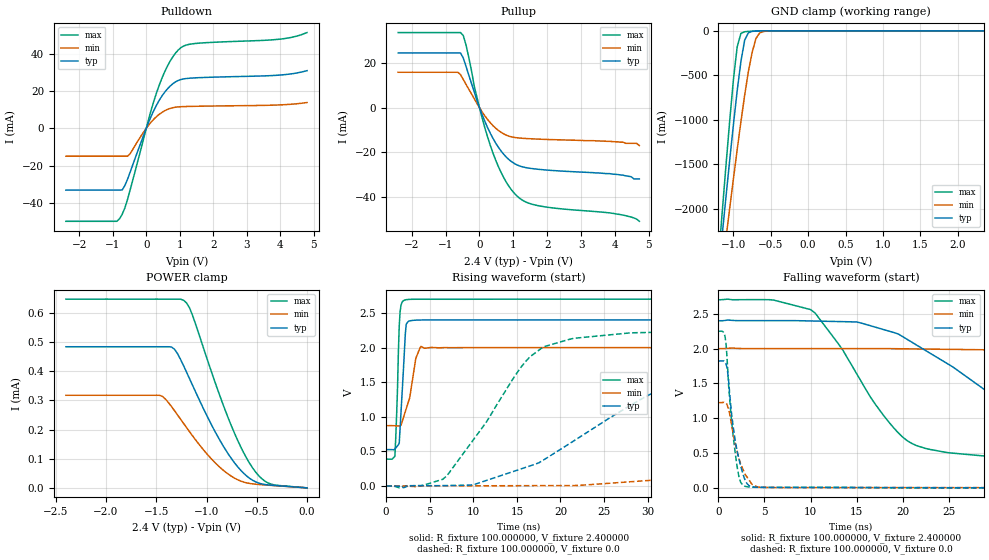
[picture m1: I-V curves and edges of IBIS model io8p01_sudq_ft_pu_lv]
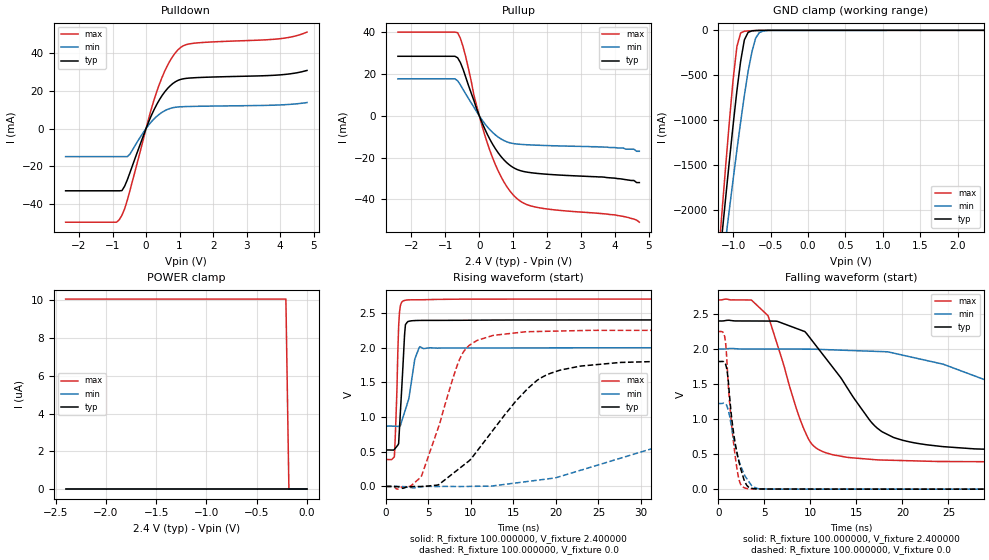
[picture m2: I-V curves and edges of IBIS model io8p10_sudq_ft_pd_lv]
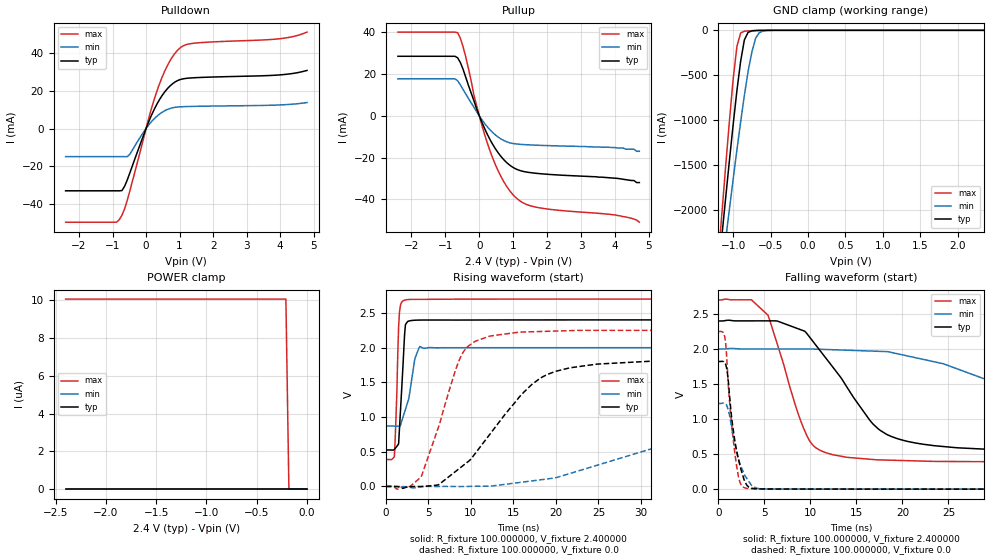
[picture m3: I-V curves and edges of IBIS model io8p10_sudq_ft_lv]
|   stm32f0_448_tssop20 IBIS Model
[IBIS ver]   4.2
[File name]  stm32f0_448_tssop20.ibs
[File Rev]   1.0
[Date]   15-5-2013
[Source] Data Created at STMicroelectronics
[Notes]   File originated from ELDO simulations.
[Disclaimer]  This information is for modeling purpose only and is
   not guaranted. The information is subject to change without
   notice.
[Copyright] Copyright 2015 STMicroelectronics Inc.
[Component] stm32f0_448_tssop20
[Manufacturer] STMicroelectronics
[Package]
| variable   typ   min   max
R_pkg   0.0   NA   NA
L_pkg   0.0H   NA   NA
C_pkg   0.0F   NA   NA
[Pin] signal_name  model_name   R_pin   L_pin   C_pin
1   BOOT0  vpp_test_hv
2   PF0   io8p_sudq_ft
3   PF1   io8p_sudq_ft
4   NRST   ioreset_tc_v33
5   VDDA   POWER
6   PA0   io8p_sudq_ft
7   PA1   io8p_sudq_ft
8   PA2   io8p_sudq_ft
9   PA3   io8p_sudq_ft
10   PA4   io8p_sudq_ft
11   PA5   io8p_sudq_ft
12   PA6   io8p_sudq_ft
13   PA7   io8p_sudq_ft
14   PB1   io8p_sudq_ft
15   VSS   GND
16   VDD   POWER
17   PA9   io8p_sudq_ft
18   PA10   io8p_sudq_ft
19   PA13   io8p_sudq_ft
20   PA14   io8p_sudq_ft
[Model Selector] io8p_sudq_ft
io8p01_sudq_ft_pd_lv  "SPEED01 2P0V, PD=40kOhm"
io8p01_sudq_ft_pu_lv  "SPEED01 2P0V, PU=40kOhm"
io8p01_sudq_ft_lv  "SPEED01 2P0V"
io8p10_sudq_ft_pd_lv  "SPEED10 2P0V, PD=40kOhm"
io8p10_sudq_ft_pu_lv  "SPEED10 2P0V, PU=40kOhm"
io8p10_sudq_ft_lv  "SPEED10 2P0V"
io8p11_sudq_ft_pd_lv  "SPEED11 2P0V, PD=40kOhm"
io8p11_sudq_ft_pu_lv  "SPEED11 2P0V, PU=40kOhm"
io8p11_sudq_ft_lv  "SPEED11 2P0V"
io8p01_sudq_ft_pd  "SPEED01, PD=40kOhm"
io8p01_sudq_ft_pu  "SPEED01, PU=40kOhm"
io8p01_sudq_ft  "SPEED01"
io8p10_sudq_ft_pd  "SPEED10, PD=40kOhm"
io8p10_sudq_ft_pu  "SPEED10, PU=40kOhm"
io8p10_sudq_ft  "SPEED10"
io8p11_sudq_ft_pd  "SPEED11, PD=40kOhm"
io8p11_sudq_ft_pu  "SPEED11, PU=40kOhm"
io8p11_sudq_ft  "SPEED11"
[Model Selector] ioreset_tc_v33
ioreset_tc_v33_pu_lv  "IORESET 2V + PU=40kOhm"
ioreset_tc_v33_nopu_lv  "IORESET 2V"
ioreset_tc_v33_pu  "IORESET + PU=40kOhm"
ioreset_tc_v33_nopu  "IORESET"
[Model Selector] vpp_test_hv
vpp_test_hv_3p3  "Input Buffer"
vpp_test_hv_2p4  "Input Buffer 2P0V"
| Models and submodels in the file (24): io8p01_sudq_ft_pd_lv (I/O), io8p01_sudq_ft_pu_lv (I/O), io8p01_sudq_ft_lv (I/O), io8p10_sudq_ft_pd_lv (I/O), io8p10_sudq_ft_pu_lv (I/O), io8p10_sudq_ft_lv (I/O), io8p11_sudq_ft_pd_lv (I/O), io8p11_sudq_ft_pu_lv (I/O), io8p11_sudq_ft_lv (I/O), io8p01_sudq_ft_pd (I/O), io8p01_sudq_ft_pu (I/O), io8p01_sudq_ft (I/O), io8p10_sudq_ft_pd (I/O), io8p10_sudq_ft_pu (I/O), io8p10_sudq_ft (I/O), io8p11_sudq_ft_pd (I/O), io8p11_sudq_ft_pu (I/O), io8p11_sudq_ft (I/O), ioreset_tc_v33_pu_lv (I/O_open_drain), ioreset_tc_v33_nopu_lv (I/O_open_drain), ioreset_tc_v33_pu (I/O_open_drain), ioreset_tc_v33_nopu (I/O_open_drain), vpp_test_hv_2p4 (Input), vpp_test_hv_3p3 (Input)
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|   Model io8p01_sudq_ft_pu_lv
[Model]  io8p01_sudq_ft_pu_lv
Model_type I/O
Polarity   Non-Inverting
Enable   Active-Low
Vinl =   0.720000V
Vinh =   1.680000V
Vmeas =  1.200000V
Cref =   50.000000pF
Rref =   100.000000M
Vref =   0.0V
C_comp   1.970100pF   1.887900pF   2.069400pF
[Temperature Range]   25.000000   0.125000k   -40.000000
[Pullup Reference]   2.400000V   2.000000V   2.700000V
[Pulldown Reference]   0.0V   0.0V   0.0V
[POWER Clamp Reference]   2.400000V   2.000000V   2.700000V
[GND Clamp Reference]   0.0V   0.0V   0.0V
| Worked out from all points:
|   slope of the pulldown table from 0 to 0.36 V, typ, clamps not added: 25.5 ohm
|   slope of the pullup table from 0 to 0.36 V, typ, clamps not added: 28.4 ohm
|   GND clamp passes 1 mA (typ) near -0.64 V on its own axis
|   rising waveform, R_fixture 100.000000, V_fixture 2.400000: 20-80 % time 497ps typ, 1.06ns min, 335ps max; typ from 0.527 V to 2.4 V
|   rising waveform, R_fixture 100.000000, V_fixture 0.0: 20-80 % time 14.6ns typ, 42.8ns min, 7.27ns max; typ from 0.001 V to 1.82 V
|   falling waveform, R_fixture 100.000000, V_fixture 2.400000: 20-80 % time 12.9ns typ, 32.5ns min, 7.06ns max; typ from 2.4 V to 0.527 V
|   falling waveform, R_fixture 100.000000, V_fixture 0.0: 20-80 % time 1.16ns typ, 1.4ns min, 913ps max; typ from 1.82 V to 0.001 V
[Pulldown]
|Voltage   I(typ)   I(min)   I(max)
-2.4V     -33.16mA   -14.98mA   -49.86mA
-880mV    -33.16mA   -14.98mA   -49.86mA
-800mV    -33.16mA   -14.98mA   -48.55mA
-640mV    -30.75mA   -14.98mA   -42.77mA
-480mV    -23.43mA   -13.57mA   -32.92mA
80mV      3.651mA    1.905mA    5.506mA
400mV     15.37mA    7.665mA    23.73mA
720mV     22.75mA    10.69mA    36.23mA
1.04V     26.18mA    11.57mA    43.27mA
1.52V     27.09mA    11.81mA    45.55mA
4V        28.55mA    12.55mA    47.81mA
4.8V      30.9mA     13.81mA    51.31mA
[Pullup]
|Voltage   I(typ)   I(min)   I(max)
-2.4V     24.57mA    15.91mA    33.73mA
-640mV    24.57mA    15.91mA    33.73mA
-480mV    22.32mA    12.71mA    32.43mA
-400mV    18.71mA    10.52mA    28.28mA
-160mV    7.421mA    4.162mA    10.02mA
0V        81fA       15.2pA     0A
320mV     -11.51mA   -6.781mA   -16.98mA
720mV     -21mA      -11.8mA    -31.53mA
1.2V      -26.24mA   -13.65mA   -40.83mA
1.76V     -27.69mA   -14.12mA   -44.07mA
3.84V     -29.6mA    -15.1mA    -47.2mA
4.72V     -32mA      -17mA      -51mA
[GND_clamp]
|Voltage   I(typ)   I(min)   I(max)
-2.4V     -9.788A    -9.782A    -9.734A
-1.2V     -2.718A    -3.02A     -2.568A
-1.15V    -2.29A     -2.675A    -2.036A
-1.1V     -1.868A    -2.333A    -1.515A
-1.05V    -1.454A    -1.995A    -1.012A
-950mV    -674.5mA   -1.337A    -180.5mA
-900mV    -345.2mA   -1.023A    -29.72mA
-850mV    -106.4mA   -726mA     -10.13mA
-750mV    -6.396mA   -244mA     -4.026mA
-700mV    -2.558mA   -88.61mA   -2.329mA
-600mV    -416uA     -7.739mA   -368uA
2.35V     0A         0A         0A
[POWER_clamp]
|Voltage   I(typ)   I(min)   I(max)
-2.4V     483.8uA    317.4uA    647uA
-1.47V    483.8uA    317.4uA    647uA
-1.32V    475.6uA    265.2uA    647uA
-1.23V    419.7uA    221.6uA    643.3uA
-1.17V    374.8uA    192.7uA    617.6uA
-1.14V    352.1uA    178.7uA    591.9uA
-840mV    147uA      62.15uA    289.6uA
-690mV    72.24uA    27.76uA    162.7uA
-540mV    25.74uA    13.55uA    67.63uA
-450mV    13.38uA    10.75uA    31.36uA
-360mV    9.231uA    8.535uA    12.97uA
0V        0A         0A         0A
[Ramp]
| variable   typ   min   max
dV/dt_r  1.09269/14.55881n   0.73353/42.71845n   1.34908/7.26325n
dV/dt_f  1.12400/12.83842n   0.67649/32.44923n   1.38689/7.04961n
R_load = 100.000000
[Rising Waveform]
R_fixture= 100.000000
V_fixture= 2.400000
V_fixture_min= 2.000000
V_fixture_max= 2.700000
|time   V(typ)   V(min)   V(max)
0s        526.5mV    872.5mV    388.6mV
1.001ns   534.8mV    870.7mV    429.3mV
1.301ns   581.8mV    869.1mV    1.401V
1.502ns   620.7mV    868.5mV    2.316V
1.602ns   841mV      868.2mV    2.522V
2.102ns   1.968V     1.038V     2.685V
2.302ns   2.337V     1.118V     2.692V
3.403ns   2.396V     1.846V     2.698V
4.004ns   2.398V     2.018V     2.698V
49.85ns   2.4V       2V         2.7V
[Rising Waveform]
R_fixture= 100.000000
V_fixture= 0.0
V_fixture_min= 0.0
V_fixture_max= 0.0
|time   V(typ)   V(min)   V(max)
0s        1.057mV    1.357mV    941.6uV
6.507ns   6.739mV    4.851mV    98.8mV
15.52ns   249.4mV    5.766mV    1.725V
18.02ns   374.6mV    6.657mV    2.009V
28.03ns   1.166V     62.6mV     2.213V
34.53ns   1.553V     120.9mV    2.23V
43.04ns   1.725V     229mV      2.248V
79.08ns   1.822V     883.8mV    2.25V
103.1ns   1.822V     1.116V     2.249V
249.2ns   1.822V     1.224V     2.25V
[Falling Waveform]
R_fixture= 100.000000
V_fixture= 2.400000
V_fixture_min= 2.000000
V_fixture_max= 2.700000
|time   V(typ)   V(min)   V(max)
0s        2.4V       2V         2.7V
10.01ns   2.397V     2V         2.56V
15.02ns   2.383V     2V         1.64V
20.02ns   2.171V     1.997V     729.2mV
29.53ns   1.353V     1.982V     451.1mV
38.04ns   762.8mV    1.926V     413.2mV
57.06ns   576.4mV    1.555V     391.8mV
84.58ns   537.8mV    1.049V     388.5mV
102.6ns   530.3mV    958.5mV    388.5mV
249.2ns   526.5mV    872.5mV    388.6mV
[Falling Waveform]
R_fixture= 100.000000
V_fixture= 0.0
V_fixture_min= 0.0
V_fixture_max= 0.0
|time   V(typ)   V(min)   V(max)
0s        1.822V     1.224V     2.25V
700.7ps   1.803V     1.224V     2.18V
800.8ps   1.785V     1.217V     2.098V
1.001ns   1.655V     1.167V     1.705V
1.401ns   1.091V     924.7mV    994.1mV
1.802ns   692.7mV    650.1mV    517.8mV
2.302ns   370.4mV    389.6mV    121.1mV
2.903ns   110.3mV    193.7mV    21.86mV
4.605ns   7.762mV    8.133mV    8.175mV
49.85ns   1.057mV    1.357mV    941.6uV
|   Model io8p10_sudq_ft_pd_lv
[Model]  io8p10_sudq_ft_pd_lv
Model_type I/O
Polarity   Non-Inverting
Enable   Active-Low
Vinl =   0.720000V
Vinh =   1.680000V
Vmeas =  1.200000V
Cref =   50.000000pF
Rref =   100.000000M
Vref =   0.0V
C_comp   1.970100pF   1.887900pF   2.069400pF
[Temperature Range]   25.000000   0.125000k   -40.000000
[Pullup Reference]   2.400000V   2.000000V   2.700000V
[Pulldown Reference]   0.0V   0.0V   0.0V
[POWER Clamp Reference]   2.400000V   2.000000V   2.700000V
[GND Clamp Reference]   0.0V   0.0V   0.0V
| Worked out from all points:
|   slope of the pulldown table from 0 to 0.36 V, typ, clamps not added: 25.5 ohm
|   slope of the pullup table from 0 to 0.36 V, typ, clamps not added: 28.4 ohm
|   GND clamp passes 1 mA (typ) near -0.64 V on its own axis
|   rising waveform, R_fixture 100.000000, V_fixture 2.400000: 20-80 % time 501ps typ, 1.06ns min, 337ps max; typ from 0.525 V to 2.4 V
|   rising waveform, R_fixture 100.000000, V_fixture 0.0: 20-80 % time 7.37ns typ, 21.8ns min, 3.53ns max; typ from 0 V to 1.82 V
|   falling waveform, R_fixture 100.000000, V_fixture 2.400000: 20-80 % time 6.27ns typ, 17.5ns min, 3.34ns max; typ from 2.4 V to 0.525 V
|   falling waveform, R_fixture 100.000000, V_fixture 0.0: 20-80 % time 1.15ns typ, 1.39ns min, 910ps max; typ from 1.82 V to 0 V
[Pulldown]
|Voltage   I(typ)   I(min)   I(max)
-2.4V     -33.16mA   -14.98mA   -49.86mA
-880mV    -33.16mA   -14.98mA   -49.86mA
-800mV    -33.16mA   -14.98mA   -48.55mA
-640mV    -30.75mA   -14.98mA   -42.76mA
-480mV    -23.43mA   -13.57mA   -32.92mA
80mV      3.651mA    1.905mA    5.506mA
400mV     15.37mA    7.665mA    23.73mA
720mV     22.75mA    10.69mA    36.23mA
1.04V     26.18mA    11.57mA    43.27mA
1.52V     27.09mA    11.81mA    45.55mA
4V        28.55mA    12.55mA    47.81mA
4.8V      30.9mA     13.81mA    51.31mA
[Pullup]
|Voltage   I(typ)   I(min)   I(max)
-2.4V     28.56mA    17.75mA    40.16mA
-720mV    28.56mA    17.75mA    40.16mA
-640mV    27.85mA    16.83mA    39.87mA
-480mV    22.39mA    12.66mA    33.22mA
-80mV     3.427mA    2.067mA    4.957mA
160mV     -6.219mA   -3.715mA   -9.137mA
320mV     -11.51mA   -6.781mA   -16.98mA
720mV     -21mA      -11.8mA    -31.53mA
1.12V     -25.77mA   -13.54mA   -39.82mA
1.76V     -27.69mA   -14.12mA   -44.07mA
4V        -29.9mA    -15.2mA    -47.5mA
4.72V     -32mA      -17mA      -51mA
[GND_clamp]
|Voltage   I(typ)   I(min)   I(max)
-2.4V     -9.788A    -9.782A    -9.734A
-1.2V     -2.718A    -3.021A    -2.568A
-1.15V    -2.29A     -2.675A    -2.036A
-1.1V     -1.868A    -2.333A    -1.515A
-1.05V    -1.454A    -1.995A    -1.012A
-950mV    -674.5mA   -1.337A    -180.6mA
-900mV    -345.2mA   -1.023A    -29.74mA
-850mV    -106.4mA   -726mA     -10.14mA
-750mV    -6.411mA   -244mA     -4.042mA
-700mV    -2.572mA   -88.62mA   -2.346mA
-600mV    -429.6uA   -7.75mA    -383.5uA
2.35V     59.77uA    46.33uA    66.89uA
[POWER_clamp]
|Voltage   I(typ)   I(min)   I(max)
-2.4V     0A         0A         10.06uA
-210mV    0A         0A         10.06uA
-180mV    0A         0A         0A
0V        0A         0A         0A
[Ramp]
| variable   typ   min   max
dV/dt_r  1.09206/7.36205n   0.73212/21.76780n   1.34880/3.52140n
dV/dt_f  1.12434/6.26286n   0.67629/17.46251n   1.38699/3.33301n
R_load = 100.000000
[Rising Waveform]
R_fixture= 100.000000
V_fixture= 2.400000
V_fixture_min= 2.000000
V_fixture_max= 2.700000
|time   V(typ)   V(min)   V(max)
0s        524.8mV    868.7mV    387.2mV
1.001ns   532.8mV    867mV      426.6mV
1.301ns   578.6mV    865.5mV    1.387V
1.502ns   616.5mV    864.9mV    2.303V
1.702ns   1.053V     875.4mV    2.602V
2.102ns   1.953V     1.031V     2.676V
2.302ns   2.331V     1.108V     2.683V
3.403ns   2.389V     1.835V     2.689V
4.004ns   2.392V     2.014V     2.689V
49.85ns   2.399V     1.999V     2.699V
[Rising Waveform]
R_fixture= 100.000000
V_fixture= 0.0
V_fixture_min= 0.0
V_fixture_max= 0.0
|time   V(typ)   V(min)   V(max)
0s        1.768nV    15.89nV    1.355nV
2.803ns   -3.26mV    -14.06mV   -1.551mV
4.204ns   -1.822mV   -2.484mV   153.2mV
6.206ns   24.43mV    -1.172mV   860.8mV
8.809ns   274.4mV    -1.373mV   1.867V
12.61ns   812.3mV    7.914mV    2.175V
17.82ns   1.532V     89.58mV    2.232V
23.02ns   1.735V     237.2mV    2.246V
50.05ns   1.82V      1.08V      2.248V
99.7ns    1.82V      1.221V     2.248V
[Falling Waveform]
R_fixture= 100.000000
V_fixture= 2.400000
V_fixture_min= 2.000000
V_fixture_max= 2.700000
|time   V(typ)   V(min)   V(max)
0s        2.399V     1.999V     2.699V
3.604ns   2.399V     1.998V     2.698V
5.405ns   2.398V     1.998V     2.475V
9.61ns    2.218V     1.997V     767.5mV
12.61ns   1.708V     1.986V     485.9mV
17.62ns   835.2mV    1.963V     416.1mV
24.42ns   606.3mV    1.782V     394.4mV
31.83ns   557.1mV    1.421V     389.7mV
47.25ns   529mV      987.2mV    387.3mV
99.7ns    524.8mV    868.7mV    387.2mV
[Falling Waveform]
R_fixture= 100.000000
V_fixture= 0.0
V_fixture_min= 0.0
V_fixture_max= 0.0
|time   V(typ)   V(min)   V(max)
0s        1.82V      1.221V     2.248V
700.7ps   1.8V       1.221V     2.179V
800.8ps   1.783V     1.214V     2.096V
1.001ns   1.653V     1.163V     1.703V
1.401ns   1.09V      921.9mV    991.5mV
1.802ns   688.2mV    647.3mV    514.6mV
2.302ns   364.8mV    386.2mV    116.7mV
2.903ns   104.8mV    188.7mV    16.24mV
4.705ns   2.13mV     3.846mV    2.055mV
49.85ns   1.768nV    15.89nV    1.355nV
|   Model io8p10_sudq_ft_lv
[Model]  io8p10_sudq_ft_lv
Model_type I/O
Polarity   Non-Inverting
Enable   Active-Low
Vinl =   0.720000V
Vinh =   1.680000V
Vmeas =  1.200000V
Cref =   50.000000pF
Rref =   100.000000M
Vref =   0.0V
C_comp   1.970100pF   1.887900pF   2.069400pF
[Temperature Range]   25.000000   0.125000k   -40.000000
[Pullup Reference]   2.400000V   2.000000V   2.700000V
[Pulldown Reference]   0.0V   0.0V   0.0V
[POWER Clamp Reference]   2.400000V   2.000000V   2.700000V
[GND Clamp Reference]   0.0V   0.0V   0.0V
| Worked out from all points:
|   slope of the pulldown table from 0 to 0.36 V, typ, clamps not added: 25.5 ohm
|   slope of the pullup table from 0 to 0.36 V, typ, clamps not added: 28.4 ohm
|   GND clamp passes 1 mA (typ) near -0.64 V on its own axis
|   rising waveform, R_fixture 100.000000, V_fixture 2.400000: 20-80 % time 501ps typ, 1.06ns min, 336ps max; typ from 0.525 V to 2.4 V
|   rising waveform, R_fixture 100.000000, V_fixture 0.0: 20-80 % time 7.32ns typ, 21.7ns min, 3.52ns max; typ from 0 V to 1.82 V
|   falling waveform, R_fixture 100.000000, V_fixture 2.400000: 20-80 % time 6.27ns typ, 18.5ns min, 3.33ns max; typ from 2.4 V to 0.525 V
|   falling waveform, R_fixture 100.000000, V_fixture 0.0: 20-80 % time 1.16ns typ, 1.4ns min, 914ps max; typ from 1.82 V to 0 V
[Pulldown]
|Voltage   I(typ)   I(min)   I(max)
-2.4V     -33.16mA   -14.98mA   -49.86mA
-880mV    -33.16mA   -14.98mA   -49.86mA
-800mV    -33.16mA   -14.98mA   -48.55mA
-640mV    -30.75mA   -14.98mA   -42.76mA
-480mV    -23.43mA   -13.57mA   -32.92mA
80mV      3.651mA    1.905mA    5.506mA
400mV     15.37mA    7.665mA    23.73mA
720mV     22.75mA    10.69mA    36.23mA
1.04V     26.18mA    11.57mA    43.27mA
1.52V     27.09mA    11.81mA    45.55mA
4V        28.55mA    12.55mA    47.81mA
4.8V      30.9mA     13.81mA    51.31mA
[Pullup]
|Voltage   I(typ)   I(min)   I(max)
-2.4V     28.57mA    17.75mA    40.17mA
-720mV    28.57mA    17.75mA    40.17mA
-640mV    27.85mA    16.83mA    39.88mA
-480mV    22.38mA    12.65mA    33.22mA
-80mV     3.427mA    2.066mA    4.957mA
160mV     -6.219mA   -3.715mA   -9.137mA
320mV     -11.51mA   -6.781mA   -16.98mA
720mV     -21mA      -11.8mA    -31.54mA
1.12V     -25.77mA   -13.54mA   -39.82mA
1.76V     -27.69mA   -14.12mA   -44.07mA
4V        -29.9mA    -15.2mA    -47.5mA
4.72V     -32mA      -17mA      -51mA
[GND_clamp]
|Voltage   I(typ)   I(min)   I(max)
-2.4V     -9.788A    -9.782A    -9.734A
-1.2V     -2.718A    -3.02A     -2.568A
-1.15V    -2.29A     -2.675A    -2.036A
-1.1V     -1.868A    -2.333A    -1.515A
-1.05V    -1.454A    -1.995A    -1.012A
-950mV    -674.5mA   -1.337A    -180.5mA
-900mV    -345.2mA   -1.023A    -29.72mA
-850mV    -106.4mA   -726mA     -10.13mA
-750mV    -6.396mA   -244mA     -4.026mA
-700mV    -2.558mA   -88.61mA   -2.329mA
-600mV    -416uA     -7.739mA   -368uA
2.35V     0A         0A         0A
[POWER_clamp]
|Voltage   I(typ)   I(min)   I(max)
-2.4V     0A         0A         10.06uA
-210mV    0A         0A         10.06uA
-180mV    0A         0A         0A
0V        0A         0A         0A
[Ramp]
| variable   typ   min   max
dV/dt_r  1.09308/7.31082n   0.73308/21.71145n   1.34964/3.51759n
dV/dt_f  1.12481/6.26349n   0.67631/18.49686n   1.38754/3.32485n
R_load = 100.000000
[Rising Waveform]
R_fixture= 100.000000
V_fixture= 2.400000
V_fixture_min= 2.000000
V_fixture_max= 2.700000
|time   V(typ)   V(min)   V(max)
0s        525.2mV    870.3mV    387.4mV
1.001ns   533.2mV    868.7mV    426.9mV
1.301ns   579.1mV    867.1mV    1.388V
1.502ns   617.1mV    866.5mV    2.304V
1.702ns   1.054V     877mV      2.604V
2.202ns   2.189V     1.072V     2.684V
2.603ns   2.379V     1.227V     2.693V
3.403ns   2.395V     1.838V     2.696V
4.004ns   2.397V     2.017V     2.696V
49.85ns   2.4V       2V         2.7V
[Rising Waveform]
R_fixture= 100.000000
V_fixture= 0.0
V_fixture_min= 0.0
V_fixture_max= 0.0
|time   V(typ)   V(min)   V(max)
0s        1.81nV     16.19nV    1.388nV
2.803ns   -3.281mV   -14.07mV   -1.578mV
4.204ns   -1.834mV   -2.504mV   153.3mV
8.809ns   274.6mV    -1.375mV   1.87V
12.21ns   748.9mV    4.656mV    2.166V
18.02ns   1.547V     92.84mV    2.232V
24.82ns   1.763V     304.5mV    2.249V
40.24ns   1.817V     861.6mV    2.249V
51.85ns   1.822V     1.107V     2.249V
99.7ns    1.822V     1.223V     2.249V
[Falling Waveform]
R_fixture= 100.000000
V_fixture= 2.400000
V_fixture_min= 2.000000
V_fixture_max= 2.700000
|time   V(typ)   V(min)   V(max)
0s        2.4V       2V         2.7V
3.604ns   2.401V     2V         2.703V
5.405ns   2.402V     2V         2.482V
9.81ns    2.189V     2V         715.2mV
14.01ns   1.448V     1.982V     453.6mV
18.22ns   786.7mV    1.963V     414.6mV
25.83ns   591.3mV    1.722V     393.9mV
36.04ns   545.2mV    1.277V     387.5mV
53.05ns   528.1mV    942.3mV    387.4mV
99.7ns    525.2mV    870.3mV    387.4mV
[Falling Waveform]
R_fixture= 100.000000
V_fixture= 0.0
V_fixture_min= 0.0
V_fixture_max= 0.0
|time   V(typ)   V(min)   V(max)
0s        1.822V     1.223V     2.249V
700.7ps   1.802V     1.222V     2.18V
800.8ps   1.785V     1.215V     2.098V
1.001ns   1.656V     1.165V     1.707V
1.401ns   1.093V     924.2mV    997.1mV
1.902ns   616.8mV    592mV      421.8mV
2.302ns   368.5mV    388.7mV    122.4mV
2.903ns   107.4mV    191.2mV    17.72mV
4.705ns   2.748mV    4.47mV     1.93mV
49.85ns   1.81nV     16.19nV    1.388nV
